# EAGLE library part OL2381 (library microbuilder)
OL2381 - Integrated UHF Transceiver (315/434/868/915 MHz)
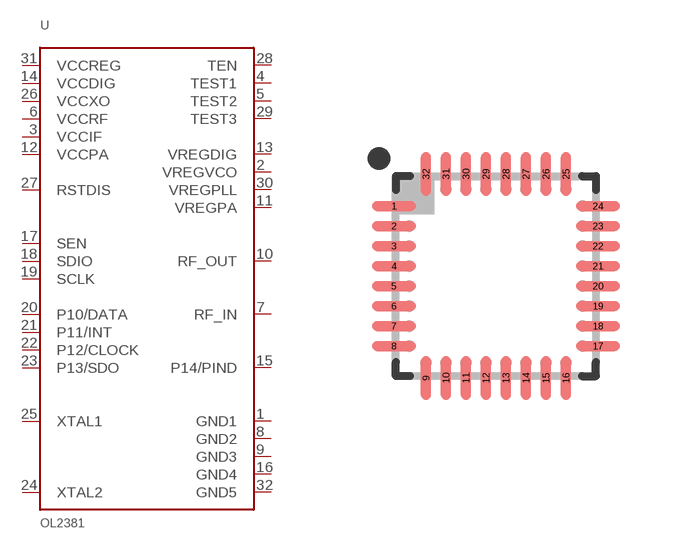
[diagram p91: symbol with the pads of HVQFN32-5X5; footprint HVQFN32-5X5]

Designator prefix U

## OL2381  [HVQFN32-5X5]
1  GND1
2  VREGVCO
3  VCCIF
4  TEST1
5  TEST2
6  VCCRF
7  RF_IN
8  GND2
9  GND3
10  RF_OUT
11  VREGPA
12  VCCPA
13  VREGDIG
14  VCCDIG
15  P14/PIND
16  GND4
17  SEN
18  SDIO
19  SCLK
20  P10/DATA
21  P11/INT
22  P12/CLOCK
23  P13/SDO
24  XTAL2
25  XTAL1
26  VCCXO
27  RSTDIS
28  TEN
29  TEST3
30  VREGPLL
31  VCCREG
32  GND5

## Footprint HVQFN32-5X5 (pad centres in mm)
HVQFN32 5x5x0.85mm (0.5mm pitch) Reference: http://ics.nxp.com/support/design/microcontrollers/smart.metering/pdf/ol2381.datasheet.pdf
smd 1.1 x 0.25: 1 -2.55,1.75; 2 -2.55,1.25; 3 -2.55,0.75; 4 -2.55,0.25; 5 -2.55,-0.25; 6 -2.55,-0.75; 7 -2.55,-1.25; 8 -2.55,-1.75; 17 2.55,-1.75; 18 2.55,-1.25; 19 2.55,-0.75; 20 2.55,-0.25; 21 2.55,0.25; 22 2.55,0.75; 23 2.55,1.25; 24 2.55,1.75
smd 0.25 x 1.1: 9 -1.75,-2.55; 10 -1.25,-2.55; 11 -0.75,-2.55; 12 -0.25,-2.55; 13 0.25,-2.55; 14 0.75,-2.55; 15 1.25,-2.55; 16 1.75,-2.55; 25 1.75,2.55; 26 1.25,2.55; 27 0.75,2.55; 28 0.25,2.55; 29 -0.25,2.55; 30 -0.75,2.55; 31 -1.25,2.55; 32 -1.75,2.55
